ORGANIZATION_BLOCK MAIN:OB1
TITLE=Ciclo automatico Sosta/Lavoro per una unità operatrice
//Simulatore: 00
//Versione: 1.0
//Data: 26/02/2002
//
//--------- Descrizione Programma ---------------------
//Il programma gestisce un ciclo di lavoro di un'unità operatrice
//mossa da un M.A.T.
//Il ciclo inizia con la pressione del pulsante SB2 (Start)
//e prosegue con tempi di lavoro (10 s) e di sosta (5 s),
//entrambi i tempi possono essere cambiati indipendentemente in
//funzioni delle esigenze.
//La gestione dei tempi di sosta e lavoro è affidata rispettivamente
//ai temporizzatori T33 e T34.
//L'arresto del ciclo è ottenuto:con la pressione del pulsante SB1
//di stop, automaticamente con l'intervento del relè termico oppure
//con la pressione del pulsante di emergenza SB3.
//Si ricorda che detta funzione di sicurezza può essere gestita solo
//da un dispositivo hardware.
//L'informazione dell'intervento viene poi riportata su un ingresso
//del PLC da un contatto (simulato da SB3) del dispositivo hardware
//di intervento.

BEGIN
NETWORK 1 //Comando Motore
//
LD Q0.0
A I0.2
O I0.1
O T34
A I0.0
A I0.4
AN T33
A I0.3
= Q0.0

NETWORK 2 //Tempo Lavoro
//
LDN T34
A Q0.0
TON T33 +100

NETWORK 3 //Set Merker Sosta
//
LD Q0.0
ED
S M0.0 1

NETWORK 4 //Reset Merker Sosta
//
LD Q0.0
EU
ON I0.0
ON I0.4
ON I0.3
R M0.0 1

NETWORK 5 //Tempo Sosta
//
LD M0.0
AN T33
TON T34 +50

NETWORK 6 //Segnalazione Relè Termico
//
LDN I0.3
= Q0.3

NETWORK 7 //Segnalazione Marcia
//
LD Q0.0
= Q0.2

NETWORK 8 //Segnalazione Arresto
//
LDN Q0.0
= Q0.1

END_ORGANIZATION_BLOCK

